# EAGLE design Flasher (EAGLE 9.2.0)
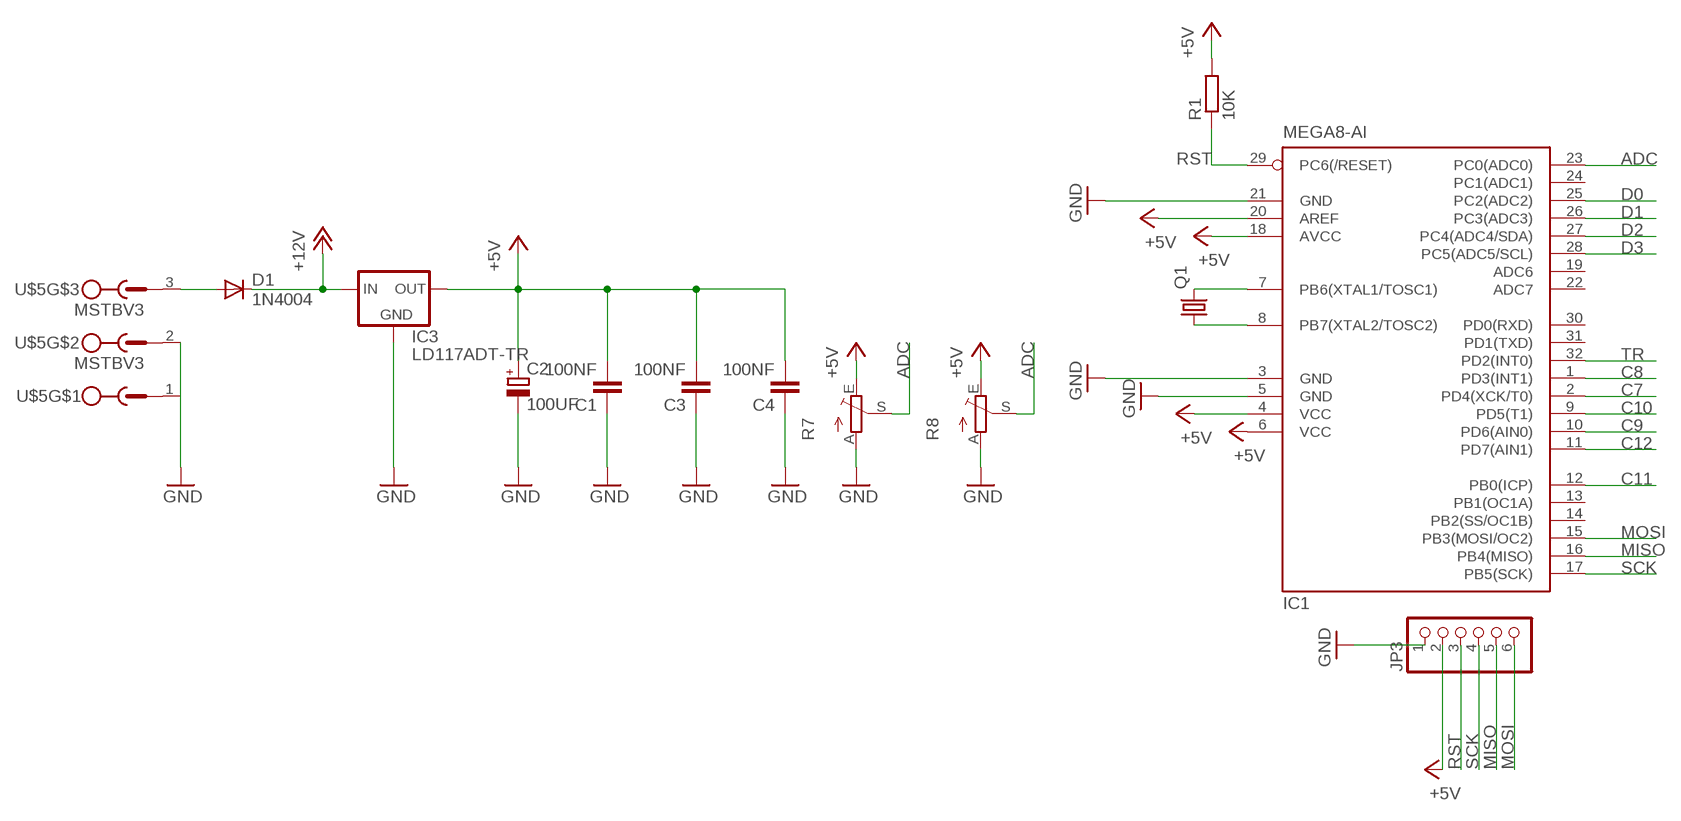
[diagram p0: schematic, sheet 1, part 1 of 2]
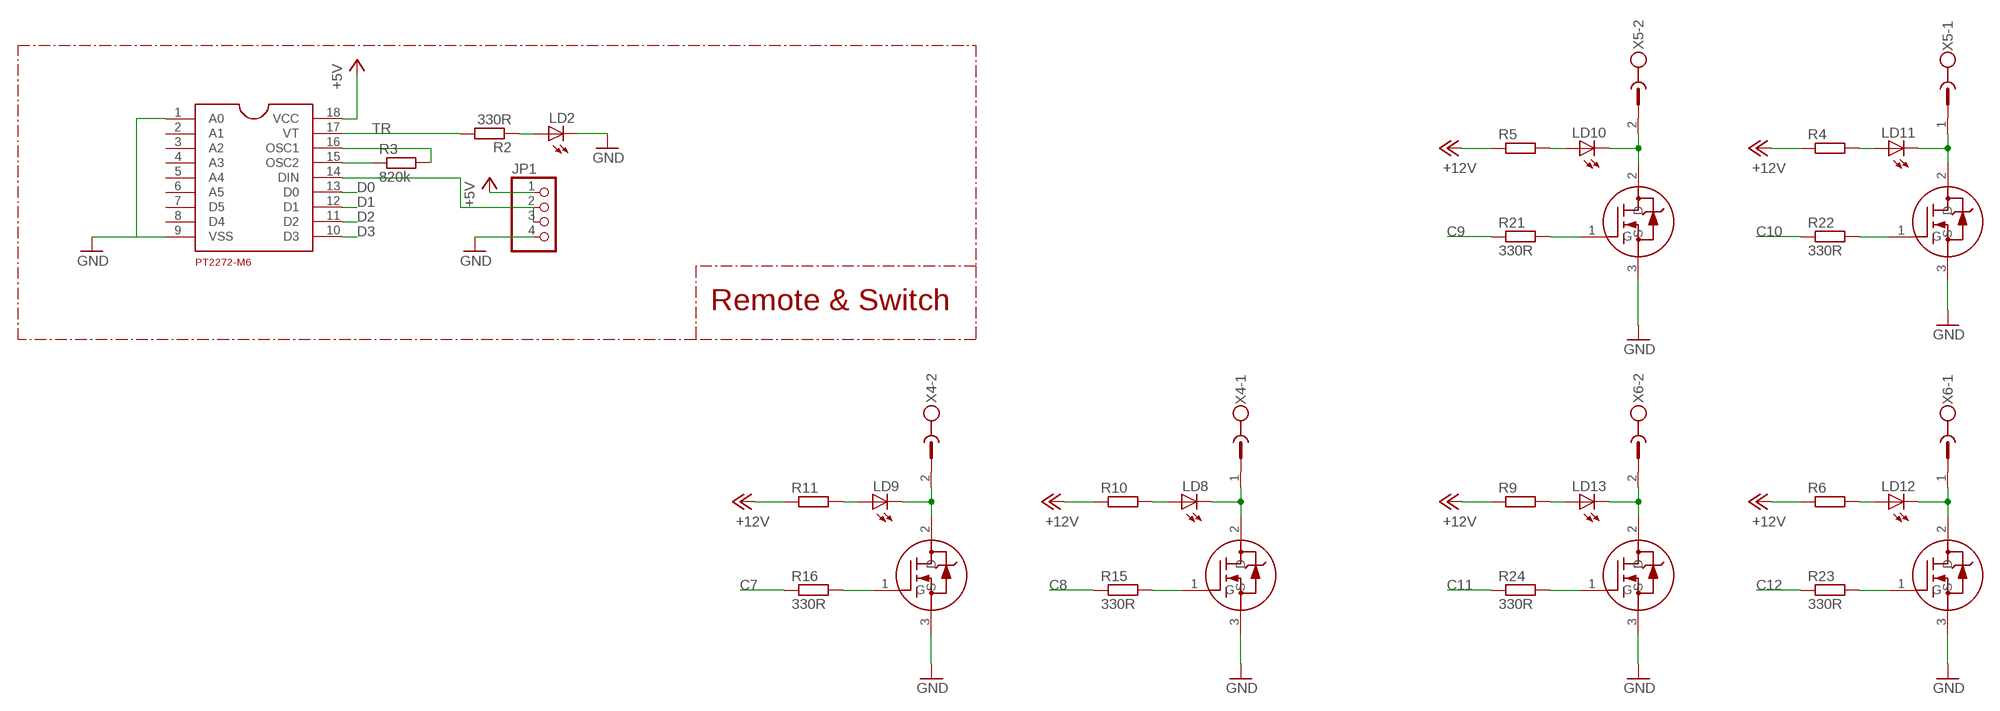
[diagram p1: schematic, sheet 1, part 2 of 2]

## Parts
C1  100NF  C-EUC0805K  [C0805K]
C2  100UF  CPOL-EUE2.5-5  [E2,5-5]
C3  100NF  C-EUC0805K  [C0805K]
C4  100NF  C-EUC0805K  [C0805K]
D1  1N4004  [DO41-10]
IC1  MEGA8-AI  [TQFP32-08]
IC3  LD117ADT-TR  [DPACK]
JP1  PINHD-1X4  [1X04]
JP3  PINHD-1X6  [1X06]
LD2  LED3MM  [LED3MM]
LD8  LED3MM  [LED3MM]
LD9  LED3MM  [LED3MM]
LD10  LED3MM  [LED3MM]
LD11  LED3MM  [LED3MM]
LD12  LED3MM  [LED3MM]
LD13  LED3MM  [LED3MM]
PT1  PT2272-M6  [18DIP]
Q1  CRYSTALHC49S  [HC49/S]
R1  10K  R-EU_0204/7  [0204/7]
R2  330R  R-EU_0204/7  [0204/7]
R3  820k  R-EU_M0805  [M0805]
R4  R-EU_M0805  [M0805]
R5  R-EU_M0805  [M0805]
R6  R-EU_M0805  [M0805]
R7  TRIM_EU-B25U  [B25U]
R8  TRIM_EU-B25P  [B25P]
R9  R-EU_M0805  [M0805]
R10  R-EU_M0805  [M0805]
R11  R-EU_M0805  [M0805]
R15  330R  R-EU_0207/10  [0207/10]
R16  330R  R-EU_0207/10  [0207/10]
R21  330R  R-EU_0207/10  [0207/10]
R22  330R  R-EU_0207/10  [0207/10]
R23  330R  R-EU_0207/10  [0207/10]
R24  330R  R-EU_0207/10  [0207/10]
U$5  MSTBV3  [MSTBV3]
U$7  20N03  [DPAK]
U$9  20N03  [DPAK]
U$10  20N03  [DPAK]
U$11  20N03  [DPAK]
U$12  20N03  [DPAK]
U$13  20N03  [DPAK]
X4  MSTBV2  [MSTBV2]
X5  MSTBV2  [MSTBV2]
X6  MSTBV2  [MSTBV2]

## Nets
+5V: C1.2 C2.+ C3.2 C4.2 IC1.4(VCC) IC1.6(VCC) IC1.18(AVCC) IC1.20(AREF) IC3.3(OUT) JP1.1 JP3.2 PT1.18(VCC) R1.2 R7.E R8.E
+12V: D1.C IC3.1(IN) R4.1 R5.1 R6.1 R9.1 R10.1 R11.1
ADC: IC1.23(PC0(ADC0)) R7.S R8.S
C7: IC1.2(PD4(XCK/T0)) R16.1
C8: IC1.1(PD3(INT1)) R15.1
C9: IC1.10(PD6(AIN0)) R21.1
C10: IC1.9(PD5(T1)) R22.1
C11: IC1.12(PB0(ICP)) R24.1
C12: IC1.11(PD7(AIN1)) R23.1
D0: IC1.25(PC2(ADC2)) PT1.13(D0)
D1: IC1.26(PC3(ADC3)) PT1.12(D1)
D2: IC1.27(PC4(ADC4/SDA)) PT1.11(D2)
D3: IC1.28(PC5(ADC5/SCL)) PT1.10(D3)
GND: C1.1 C2.- C3.1 C4.1 IC1.3(GND) IC1.5(GND) IC1.21(GND) IC3.2(GND) JP1.4 JP3.1 LD2.K(C) PT1.1(A0) PT1.9(VSS) R7.A R8.A U$5.1 U$5.2 U$7.3(S) U$9.3(S) U$10.3(S) U$11.3(S) U$12.3(S) U$13.3(S)
MISO: IC1.16(PB4(MISO)) JP3.5
MOSI: IC1.15(PB3(MOSI/OC2)) JP3.6
N$1: PT1.15(OSC2) R3.1
N$2: D1.A U$5.3
N$3: IC1.8(PB7(XTAL2/TOSC2)) Q1.1
N$4: IC1.7(PB6(XTAL1/TOSC1)) Q1.2
N$9: PT1.16(OSC1) R3.2
N$19: LD8.K(C) U$9.2(D) X4.1
N$21: R16.2 U$7.1(G)
N$22: R15.2 U$9.1(G)
N$26: LD8.A R10.2
N$27: LD9.A R11.2
N$28: LD9.K(C) U$7.2(D) X4.2
N$29: LD10.K(C) U$10.2(D) X5.2
N$30: LD11.K(C) U$12.2(D) X5.1
N$31: LD12.K(C) U$13.2(D) X6.1
N$32: R21.2 U$10.1(G)
N$33: R24.2 U$11.1(G)
N$34: R23.2 U$13.1(G)
N$35: R22.2 U$12.1(G)
N$36: LD10.A R5.2
N$37: LD11.A R4.2
N$38: LD12.A R6.2
N$39: LD13.A R9.2
N$40: LD13.K(C) U$11.2(D) X6.2
N$52: LD2.A R2.1
N$53: JP1.2 JP1.3 PT1.14(DIN)
RST: IC1.29(PC6(/RESET)) JP3.3 R1.1
SCK: IC1.17(PB5(SCK)) JP3.4
TR: IC1.32(PD2(INT0)) PT1.17(VT) R2.2
Unconnected: IC1.13(PB1(OC1A)) IC1.14(PB2(SS/OC1B)) IC1.19(ADC6) IC1.22(ADC7) IC1.24(PC1(ADC1)) IC1.30(PD0(RXD)) IC1.31(PD1(TXD)) PT1.2(A1) PT1.3(A2) PT1.4(A3) PT1.5(A4) PT1.6(A5) PT1.7(D5) PT1.8(D4)

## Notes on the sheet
- Remote & Switch

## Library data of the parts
C1 C3 C4 = rcl:C-EU: CAPACITOR, European symbol
C2 = rcl:CPOL-EU: POLARIZED CAPACITOR, European symbol
D1 = diode:1N4004: DIODE
IC1 = atmel:MEGA8: MICROCONTROLLER 8 Kbytes FLASH, 1 kbytes SRAM, 512 bytes EEPROM, USART, 6-channel 10 bit ADC, 2-channel 8 bit ADC Pin compatible with Atmega48, ATMega88, ATMega168 Source: avr.lbr; MPN: ATMEGA8-16AU; OC_FARNELL: 9171371; OC_NEWARK: 73M8863
IC3 = v-reg:LD117A?*: Low drop fixed and adjustable positive voltage regulators 1 A Source: http://www.st.com/stonline/products/literature/ds/7194/ld1117axx.pdf
JP1 = pinhead:PINHD-1X4: PIN HEADER
JP3 = pinhead:PINHD-1X6: PIN HEADER
LD2 LD8-LD13 = led:LED: LED
PT1 = PT:PT2272-M6: DIP18
Q1 = crystal:CRYSTAL: CRYSTAL; OC_FARNELL: 1667008; OC_NEWARK: unknown
R1 R3-R6 R9-R11 R15 R16 R21-R24 = rcl:R-EU_: RESISTOR, European symbol
R2 = resistor:R-EU_: RESISTOR, European symbol
R7 R8 = pot:TRIM_EU-: POTENTIOMETER
U$5 = con-phoenix-500:MSTBV3
U$7 U$9-U$13 = 20n03:20N03
X4-X6 = con-phoenix-500:MSTBV2: PHOENIX; OC_FARNELL: unknown; OC_NEWARK: unknown

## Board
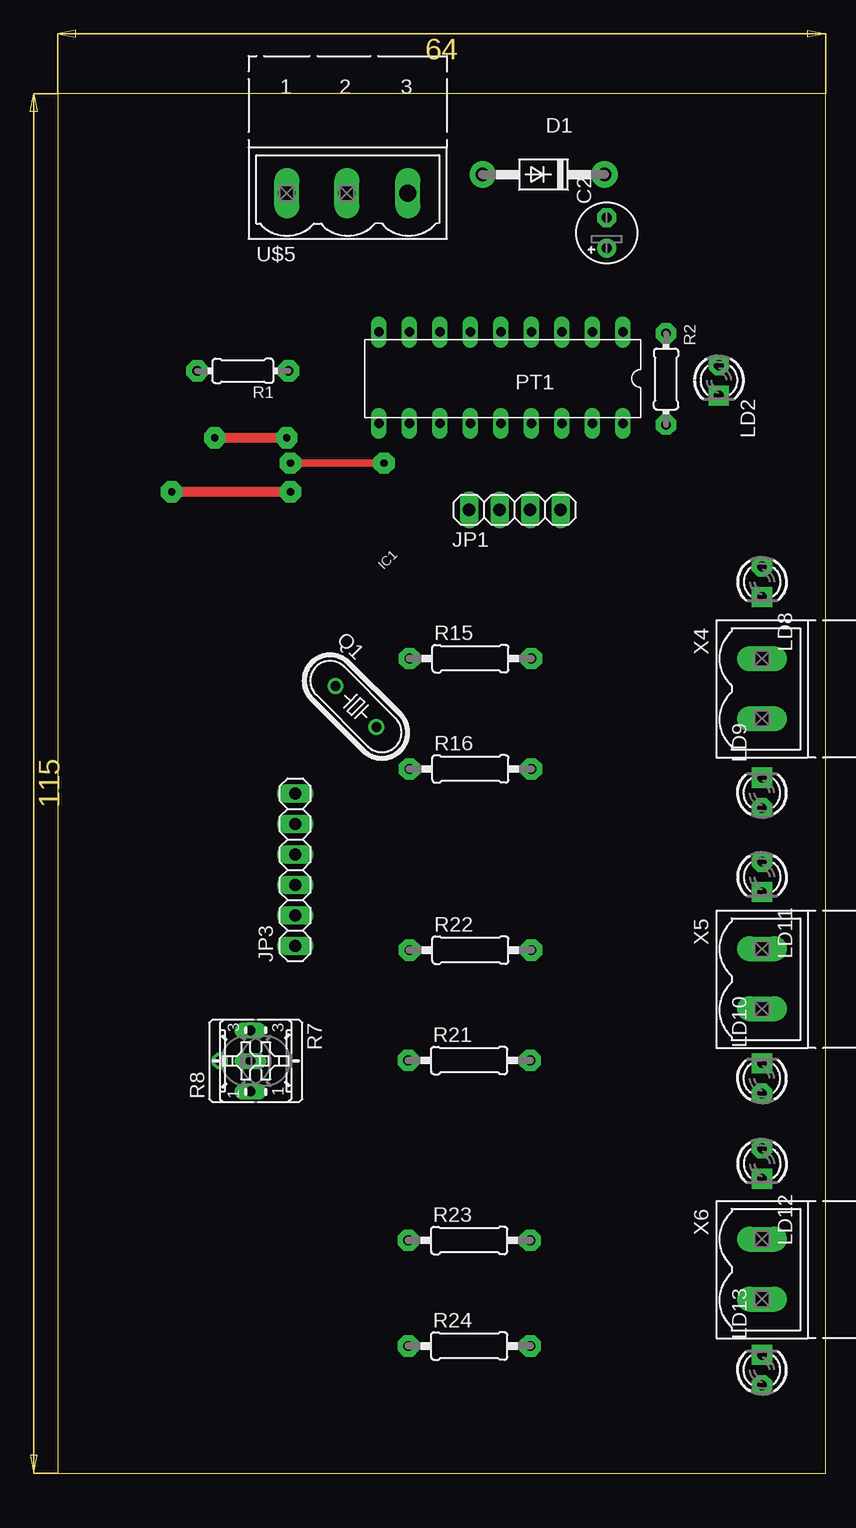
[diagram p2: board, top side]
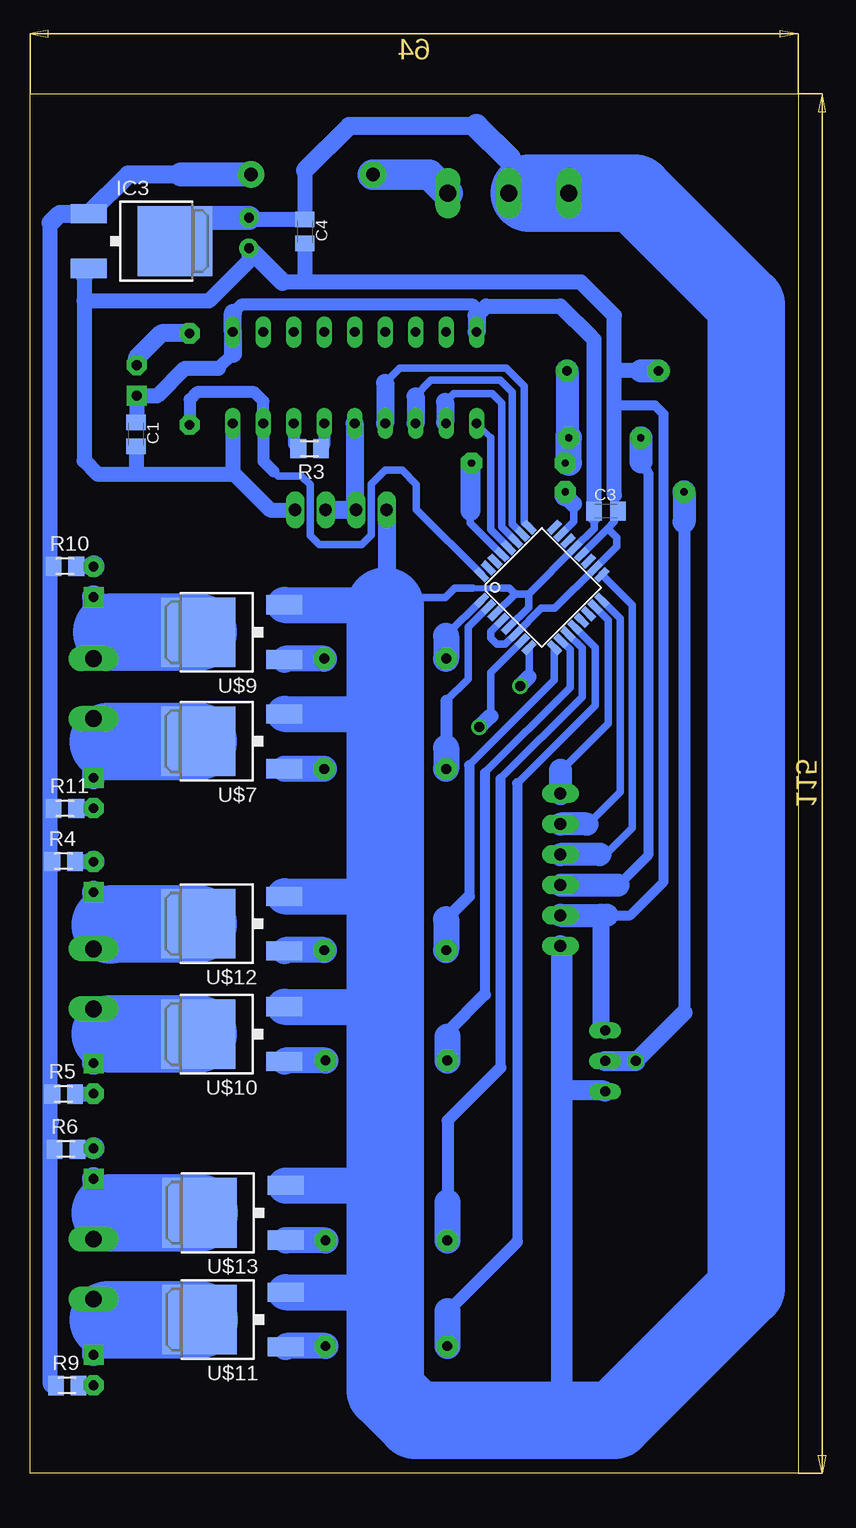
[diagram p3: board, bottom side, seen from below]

Size 66.3 x 120.3 mm. Coordinates in mm from the lower left corner, seen from the top.
Outline: 2.3,0 66.3,0 66.3,115 2.3,115 2.3,0
Copper layers (1*16): Top 0.035mm / dielectric 1.5mm / Bottom 0.035mm
Design rules "default": minimum track width 10mil, minimum drill 24mil, track to track 8mil, track to pad 8mil, pad to pad 8mil, via to via 8mil, smd to smd 8mil, copper to edge 40mil, drill to drill 8mil, minimum pad ring 10mil, minimum via ring 8mil, stop-mask expansion 4mil, vias tented up to drill 0mil, thermal gap 10mil

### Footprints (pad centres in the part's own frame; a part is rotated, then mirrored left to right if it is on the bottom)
C0805K = smd 1.3 x 1.6: 1 -1,0; 2 1,0
E2,5-5 = drill 0.813 pad 1.6: + -1.27,0 | drill 0.813 pad 1.6 octagon: - 1.27,0
DO41-10 = drill 1.118 pad 2.184: A 5.08,0; C -5.08,0
TQFP32-08 = smd 1.27 x 0.559: 1 -4.293,2.8; 2 -4.293,2; 3 -4.293,1.2; 4 -4.293,0.4; 5 -4.293,-0.4; 6 -4.293,-1.2; 7 -4.293,-2; 8 -4.293,-2.8; 17 4.293,-2.8; 18 4.293,-2; 19 4.293,-1.2; 20 4.293,-0.4; 21 4.293,0.4; 22 4.293,1.2; 23 4.293,2; 24 4.293,2.8 | smd 0.559 x 1.27: 9 -2.8,-4.293; 10 -2,-4.293; 11 -1.2,-4.293; 12 -0.4,-4.293; 13 0.4,-4.293; 14 1.2,-4.293; 15 2,-4.293; 16 2.8,-4.293; 25 2.8,4.293; 26 2,4.293; 27 1.2,4.293; 28 0.4,4.293; 29 -0.4,4.293; 30 -1.2,4.293; 31 -2,4.293; 32 -2.8,4.293
DPACK = smd 1.6 x 3: 1 -2.28,-4.8; 3 2.28,-4.8 | smd 5.8 x 6.2: 2 0,2.38
1X04 = drill 1.016 long: 1 -3.81,0; 2 -1.27,0; 3 1.27,0; 4 3.81,0
1X06 = drill 1.016 long: 1 -6.35,0; 2 -3.81,0; 3 -1.27,0; 4 1.27,0; 5 3.81,0; 6 6.35,0
LED3MM = drill 0.813 pad 1.676 octagon: A -1.27,0 | drill 0.813 pad 1.676 square: K 1.27,0
18DIP = drill 0.8 long: 1 -10,-4.12; 2 -7.46,-4.12; 3 -4.92,-4.12; 4 -2.38,-4.12; 5 0.16,-4.12; 6 2.7,-4.12; 7 5.24,-4.12; 8 7.78,-4.12; 9 10.32,-4.12; 10 10.32,3.5; 11 7.78,3.5; 12 5.24,3.5; 13 2.7,3.5; 14 0.16,3.5; 15 -2.38,3.5; 16 -4.92,3.5; 17 -7.46,3.5; 18 -10,3.5
HC49/S = drill 0.813: 1 -2.413,0; 2 2.413,0
0204/7 = drill 0.813 pad 1.778 octagon: 1 -3.81,0; 2 3.81,0
0204/7' = drill 0.813 pad 1.676 octagon: 1 -3.81,0; 2 3.81,0
M0805 = smd 1.3 x 1.6: 1 -0.95,0; 2 0.95,0
B25U = drill 0.813 long: A 2.54,-0.889; E -2.54,-0.889; S 0,-0.889
B25P = drill 0.813 octagon: A -2.54,0; E 2.54,0; S 0,2.54
0207/10 = drill 0.813 pad 1.778 octagon: 1 -5.08,0; 2 5.08,0
MSTBV3 = drill 1.397 long: 1 -2.5,0; 2 2.5,0; 3 7.58,0
DPAK = smd 1.6 x 3: 1 -2.28,-4.8; 3 2.28,-4.8 | smd 5.8 x 6.2: 2 0,2.38
MSTBV2 = drill 1.397 long: 1 -2.5,0; 2 2.5,0

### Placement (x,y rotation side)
C1  57.46,86.6 270 bottom
C2  48.06,103.38 90 top
C3  18.3,80.2 0 bottom
C4  43.4,103.5 270 bottom
D1  42.8,108.25 180 top
IC1  23.65,73.83 45 bottom
IC3  56.6,102.7 270 bottom
JP1  40.4,80.3 180 top
JP3  22.1,50.3 90 top
LD2  57.4,91.1 270 top
LD8  61,74.3 270 top
LD9  61,56.7 90 top
LD10  61,32.9 90 top
LD11  61,49.7 270 top
LD12  61,25.8 270 top
LD13  61,8.6 90 top
PT1  39.4,91 180 top
Q1  27.16,63.9 315 top
R1  17.74,91.88 180 top
R2  330R  [0204/7']  53,91.2 270 top
R3  43,85.4 180 bottom
R4  63.5,51 0 bottom
R5  63.5,31.6 0 bottom
R6  63.3,27 0 bottom
R7  19.26,34.36 270 top
R8  18.37,34.36 90 top
R9  63.2,7.3 0 bottom
R10  63.4,75.6 0 bottom
R11  63.4,55.4 0 bottom
R15  36.7,67.9 0 top
R16  36.7,58.7 0 top
R21  36.6,34.4 0 top
R22  36.7,43.6 0 top
R23  36.6,19.4 0 top
R24  36.6,10.6 0 top
U$5  23.9,106.7 0 top
U$7  49.9,61 90 bottom
U$9  49.9,70.1 90 bottom
U$10  49.9,36.6 90 bottom
U$11  49.8,12.8 90 bottom
U$12  49.9,45.8 90 bottom
U$13  49.8,21.7 90 bottom
X4  61,65.4 270 top
X5  61,41.2 270 top
X6  61,17 270 top

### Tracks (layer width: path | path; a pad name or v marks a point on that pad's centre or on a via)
+5V
  Bottom 0.61: IC1.4 27.9,70.15 27.9,69.6 27.4,69.1 26.69,69.1 IC1.6 23.69,72.1 22.55,72.1 IC1.18 17.4,77.25 17.4,78 18.11,78.71 18.21,78.71 | IC1.20 18.21,78.71 | 18.21,78.71 17.6,79.32 17.6,79.9 | 17.6,79.9 17.6,81.5 | C3.2 17.6,79.9
  Bottom 0.813: 18.2,46.5 16.3,46.5 13.5,49.3 13.5,88.3 14.2,89 17.6,89
  Bottom 1.016: R8.E
  Bottom 1.27: 17.6,81.5 17.6,89 17.6,92 | 17.6,92 17.6,96.5 20.4,99.3 43.5,99.3 | 15.4,91.9 17.5,91.9 17.6,92 | 43.5,99.3 45.25,99.3 | 48.09,102.08 C2.+ 48.06,101.04 51.4,97.7 61.8,97.7 | C4.2 43.4,99.4 43.5,99.3 | PT1.18 49.4,83.4 | JP1.1 46.3,80.3 49.4,83.4 | 61.8,99.9 61.8,97.7 | 61.8,97.7 61.8,84.4 60.7,83.3 57.5,83.3 | 57.5,83.3 49.5,83.3 49.4,83.4 | C1.2 57.46,83.34 57.5,83.3
  Bottom 1.422: R8.E 18.7,37.23 18.7,46.49
  Bottom 1.5: C2.+ 45.25,99.3 | IC3.3 61.4,100.3 61.8,99.9
  Bottom 1.93: JP3.2 18.7,46.49 18.21,46.49 18.2,46.5 | R1.2 15.38,91.88 15.4,91.9
+12V
  Bottom 1.27: 64.6,27.1 64.6,7.4 64.5,7.3 R9.1 | 64.6,27.1 64.6,29.2 | 64.6,29.2 64.6,31.7 | 64.6,31.7 64.6,51.1 | 64.6,51.1 64.6,53.4 | 64.6,53.4 64.6,55.4 | 64.6,55.4 64.6,75.4 | 64.6,75.4 64.6,104.2 | 64.5,29.3 64.6,29.2 | 64.5,53.3 64.6,53.4 | R10.1 64.55,75.4 64.6,75.4 | R11.1 64.6,55.4 | R4.1 64.5,51 64.6,51.1 | R5.1 64.5,31.6 64.6,31.7 | R6.1 64.5,27 64.6,27.1
  Bottom 1.5: 53.73,108.25 58.13,108.25 IC3.1 63.82,104.98 64.6,104.2
  Bottom 2: D1.C 53.73,108.25
ADC  (via drill 0.6 pad 1.78)
  Top 0.813: v21.7,81.8 v11.8,81.8
  Bottom 0.61: IC1.23 21,79.31 21,80.8
  Bottom 1.016: 11.8,79.3 11.8,38.38
  Bottom 1.422: 21,80.8 21.7,81.5 | 11.8,38.38 R8.S
  Bottom 1.676: R7.S R8.S
  Bottom 1.778: 21.7,81.5 v21.7,81.8
  Bottom 1.93: v11.8,81.8 11.8,79.3
C7
  Bottom 0.61: IC1.2 29.8,70.51 29.8,66.2 31.6,64.4
  Bottom 1.016: 31.6,64.4 31.6,60.5
  Bottom 1.93: 31.6,60.5 31.62,60.48
  Bottom 2.184: 31.62,60.48 R16.1
C8
  Bottom 0.61: IC1.1 31.6,69.84 31.6,69.8
  Bottom 1.93: 31.6,69.8 31.62,69.78
  Bottom 2.184: 31.62,69.78 R15.1
C9
  Bottom 0.61: IC1.10 21.3,68.65 21.3,65.5 28.4,58.4 | 31.5,36.8 31.5,36.4
  Bottom 0.813: 28.4,58.4 28.4,39.9
  Bottom 1.016: 31.5,36.8 28.4,39.9
  Bottom 1.93: 31.5,36.4 31.52,36.38
  Bottom 2.184: 31.52,36.38 R21.1
C10
  Bottom 0.61: 29.7,59.01 22.6,66.11 IC1.9
  Bottom 0.813: 29.7,59.01 29.7,48.1
  Bottom 1.016: 31.6,46.2 29.7,48.1
  Bottom 1.93: 31.6,46.2 31.62,46.18
  Bottom 2.184: 31.62,46.18 R22.1
C11
  Bottom 0.61: IC1.12 19.2,68.81 19.2,64 25.7,57.5
  Bottom 0.813: 25.7,57.5 25.7,19.3
  Bottom 1.016: 31.5,13.5 25.7,19.3
  Bottom 2.184: 31.5,13.5 31.52,13.48 R24.1
C12
  Bottom 0.61: IC1.11 20.3,68.78 20.3,64.7 27.1,57.9
  Bottom 0.813: 27.1,57.9 27.1,33.8
  Bottom 1.016: 27.1,33.8 31.5,29.4 31.5,22.6
  Bottom 2.184: 31.5,22.6 31.52,22.58 R23.1
D0
  Bottom 0.61: IC1.25 25.1,79.24 25.1,90.6 26.6,92.1 35.5,92.1 36.7,90.9
  Bottom 1.5: 36.7,90.9 PT1.13
D1
  Bottom 0.61: IC1.26 26.1,79.1 26.1,90.1 27.1,91.1 32.9,91.1 34.2,89.8 34.16,89.76
  Bottom 1.5: 34.16,89.76 PT1.12
D2
  Bottom 0.61: IC1.27 27,78.87 27,89.2 27.8,90 31,90 31.7,89.3 | 31.7,87.58 PT1.11
  Bottom 1.5: 31.7,89.3 31.7,87.58
D3
  Bottom 0.508: 27.9,86.32 PT1.10
  Bottom 0.61: IC1.28 27.9,78.64 27.9,86.32
GND
  Bottom 0.508: 29.4,73.8 27,73.8
  Bottom 0.61: 24.75,73.3 25.88,73.3 | IC1.3 25.88,73.3 | IC1.5 24.75,72.17 24.75,73.3 | 24.75,73.3 IC1.21 19.3,78.75 19.3,79.7 | 36.59,73 31.7,73 30.9,73.8 29.4,73.8 | 27,73.8 26.38,73.8 25.88,73.3
  Bottom 0.813: 19.45,94.65 19.5,94.7 arc90 19.3,94.5
  Bottom 1.016: R8.A | 49.4,96.7 48.7,97.4 29.36,97.4 29.08,97.12 29.08,96.5 | 49.4,93.3 50.6,92.1
  Bottom 1.27: 19.3,79.7 C3.1 19.3,94.5 | 19.5,94.7 22.1,97.3 28.28,97.3 29.08,96.5 | C2.- 47.91,104.5 C4.1 43.4,108.6 | 26.4,109.6 U$5.2 | 50.6,92.1 53.4,92.1 55.7,89.8 57.37,89.8 LD2.K 57.4,87.66 C1.1
  Bottom 1.5: JP1.4 36.59,73 36.59,72.41 36.7,72.3 | 49.4,96.7 PT1.1 49.4,93.3 | 29.08,96.5 PT1.9 | 29.1,112.3 39.7,112.3 43.4,108.6 | IC3.2 54.22,104.42 53.99,104.65
  Bottom 1.676: R8.A 18.45,31.9 22,31.9
  Bottom 1.778: JP3.1 22,43.85 22,31.9 22,4.4
  Bottom 2: 53.99,104.65 C2.- | 26.4,109.6 29.1,112.3
  Bottom 2.54: 24.7,106.7 U$5.2
  Bottom 3: U$11.3 36.88,15.08 36.7,14.9 | U$13.3 36.88,23.98 36.7,23.8 | U$10.3 36.38,38.88 36.2,38.7 36.4,38.7 36.7,39 | U$12.3 36.82,48.08 36.7,48.2 | U$7.3 36.82,63.28 36.7,63.4 | U$9.3 36.78,72.38 36.7,72.3
  Bottom 6.452: 36.7,72.3 36.7,63.4 36.7,48.2 36.7,39 36.7,23.8 36.7,14.9 36.7,6.9 34.2,4.4 22,4.4 17.6,4.4 6.6,15.4 6.6,97.4 15.9,106.7 U$5.1 24.7,106.7
MISO
  Bottom 0.61: IC1.16 17.1,71.24 17.1,56.8 19.8,54.1 19.9,54.1
  Bottom 1.93: 19.9,54.1 19.91,54.11 JP3.5
MOSI
  Bottom 0.61: IC1.15 18.1,71.1 18.1,62.5 22,58.6 22.1,58.6
  Bottom 1.93: 22.1,58.6 JP3.6
N$1
  Bottom 1.016: PT1.15 41.78,85.67 R3.1
N$2
  Bottom 2.54: D1.A 33.03,108.25 U$5.3
N$3
  Bottom 0.61: IC1.8 24.71,66.41 24.7,66.4
  Bottom 1.27: 24.7,66.4 25.45,65.65 Q1.1
N$4
  Bottom 0.61: IC1.7 27.9,66.75 27.9,63.1
  Bottom 1.27: 27.9,63.1 27.96,63.1 Q1.2
N$9
  Bottom 1.016: PT1.16 44.32,85.77 R3.2
N$19
  Bottom 1.93: X4.1 61,68.6 59.5,70.1 61,71.6 LD8.K
  Bottom 6.452: U$9.2 59.5,70.1
N$21
  Bottom 2.184: R16.2 45.08,58.7 U$7.1
N$22
  Bottom 2.184: R15.2 45.02,67.9 U$9.1
N$26
  Bottom 1.27: R10.2 60.97,75.6
  Bottom 1.778: 60.97,75.6 LD8.A
N$27
  Bottom 1.27: R11.2 61.03,55.4 LD9.A
N$28
  Bottom 1.93: LD9.K 61,59.8 59.8,61 61,62.2 X4.2
  Bottom 6.452: U$7.2 59.8,61
N$29
  Bottom 1.93: LD10.K 61,35.2 59.6,36.6 61,38 X5.2
  Bottom 6.452: U$10.2 59.6,36.6
N$30
  Bottom 1.93: X5.1 61,44.3 59.6,45.7 | LD11.K 61,47.3 59.5,45.8
  Bottom 6.452: U$12.2 59.5,45.8 59.6,45.7
N$31
  Bottom 1.93: X6.1 61,20.3 59.6,21.7 61,23.1 LD12.K
  Bottom 6.452: U$13.2 59.6,21.7
N$32
  Bottom 2.184: R21.2 45.02,34.4 U$10.1
N$33
  Bottom 2.184: R24.2 44.92,10.6 U$11.1
N$34
  Bottom 2.184: R23.2 44.98,19.4 U$13.1
N$35
  Bottom 2.184: R22.2 45.02,43.6 U$12.1
N$36
  Bottom 1.27: R5.2 61.03,31.6 LD10.A
N$37
  Bottom 1.27: R4.2 60.97,51
  Bottom 1.778: 60.97,51 LD11.A
N$38
  Bottom 1.27: R6.2 61.07,27 60.97,27.1
  Bottom 1.778: 60.97,27.1 LD12.A
N$39
  Bottom 1.27: R9.2 61.03,7.3 LD13.A
N$40
  Bottom 1.93: LD13.K 61,11.6 59.8,12.8 61,14 X6.2
  Bottom 6.452: U$11.2 59.8,12.8
N$52
  Bottom 1.5: R2.1 55.36,95.01 57.4,92.97 LD2.A
N$53
  Bottom 1.5: PT1.14 39.24,80.41 JP1.3 JP1.2
RST  (via drill 0.6 pad 1.78)
  Top 0.61: v29.5,84.2 v21.7,84.2
  Top 0.813: v21.4,86.3 v15.4,86.3
  Bottom 0.61: IC1.29 29.6,79.21 29.6,80.2
  Bottom 0.813: v21.7,84.2 21.4,84.2 | 17.3,49 14.8,51.5 14.8,83.4 15.4,84 15.4,84.3 | 22.07,49 JP3.3
  Bottom 1.676: v29.5,84.2 29.6,84.1 29.6,80.2
  Bottom 1.93: 17.3,49 22.07,49 | v15.4,86.3 15.4,84.3 | R1.1 21.55,86.45 v21.4,86.3
  Bottom 2.184: 21.4,84.2 v21.4,86.3
SCK
  Bottom 0.61: IC1.17 16.1,72.35 16.1,53.8 18.3,51.6 18.8,51.6
  Bottom 1.93: 18.8,51.6 18.83,51.57 JP3.4
TR
  Bottom 0.61: IC1.32 34.1,80.32 34.1,82.4 35.3,83.6 36.7,83.6 37.86,82.44 37.86,79.01 37.85,79 37.85,78.2 38.65,77.4 42.2,77.4 42.94,78.14 42.94,82.39 43.68,83.13 45.63,83.13 46,83.5
  Bottom 1.016: R2.2 53,89.5 52.4,90.1 47.6,90.1 46.86,89.36 PT1.17 46.86,84.36 46,83.5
